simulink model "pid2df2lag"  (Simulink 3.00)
settings: Solver=ode45  SolverMode=SingleTasking  StartTime=0.0  StopTime=10.0  MaxStep=st_size  RelTol=1e-5  AbsTol=1e-6
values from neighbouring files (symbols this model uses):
  d_through_p = get(MAIN_MENU(19),'Value')    [cback.m]    (also in imcmenu.m = 0)
  Disturb = Setpoint    [mimo_MSF1DF_sim.m]    (also in mimo_MSF2DF_sim.m)
  Satlb = temp1    [cback.m]    (also in imcmenu.m = str2num(satlbs))
  Satub = temp1    [cback.m]    (also in imcmenu.m = str2num(satubs))
  Setpoint = zeros(1,n)    [mimo_MSF1DF_sim.m]    (also in mimo_MSF2DF_sim.m)
undefined symbols (not defined in the file or in its folder): a1, a2, b1, b2, denPd, denPs, keps, numPd, numPs, Pre_fil_den, Pre_fil_num
libraries: MIMO_lib x1

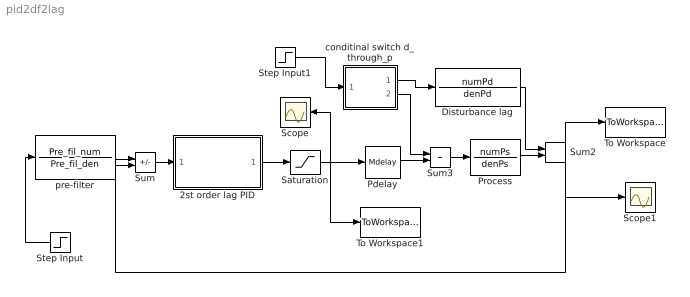
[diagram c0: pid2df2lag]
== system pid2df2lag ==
  2st order lag PID : Subsystem
  Disturbance lag : TransferFcn  Numerator=numPd  Denominator=denPd
  Pdelay : MIMO_lib/Mdelay  Mdelay=Pdelay
  Process : TransferFcn  Numerator=numPs  Denominator=denPs
  Saturation : Saturate  UpperLimit=Satub  LowerLimit=Satlb
  Scope : Scope
  Scope1 : Scope
  Step Input : Step  Orientation=left  Time=0  Before=0  After=Setpoint  SampleTime=0
  Step Input1 : Step  Time=0  Before=0  After=Disturb  SampleTime=0
  Sum : Sum  Inputs=+-  SaturateOnIntegerOverflow=on
  Sum2 : Sum  Inputs=++  SaturateOnIntegerOverflow=on
  Sum3 : Sum  Inputs=++  SaturateOnIntegerOverflow=on
  To Workspace : ToWorkspace  VariableName=simout  SampleTime=-1  SaveFormat=Matrix
  To Workspace1 : ToWorkspace  VariableName=effort  SampleTime=-1  SaveFormat=Matrix
  conditinal switch d_through_p : Subsystem  Description=pass input signal through out1 if condition is true.
  pre-filter : TransferFcn  Numerator=Pre_fil_num  Denominator=Pre_fil_den
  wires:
  Disturbance lag/1 -> Sum2/1
  Sum/1 -> 2st order lag PID/1(In1)
  pre-filter/1 -> Sum/1
  Step Input/1 -> pre-filter/1
  2st order lag PID/1(Out1) -> Saturation/1
  Step Input1/1 -> conditinal switch d_through_p/1(In)
  conditinal switch d_through_p/1(Out2) -> Disturbance lag/1
  conditinal switch d_through_p/2(Out1) -> Sum3/1
  Pdelay/1 -> Sum3/2
  Sum3/1 -> Process/1
  Process/1 -> Sum2/2
  Sum2/1 -> Sum/2, To Workspace/1, Scope1/1
  Saturation/1 -> Pdelay/1, Scope/1, To Workspace1/1

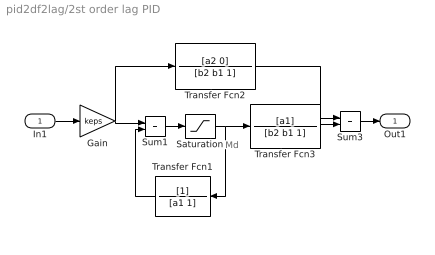
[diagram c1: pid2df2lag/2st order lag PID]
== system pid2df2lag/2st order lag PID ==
  note: Md
  In1 : Inport  Port=1  PortWidth=-1  SampleTime=-1  DataType=auto
  Gain : Gain  Gain=keps  SaturateOnIntegerOverflow=on
  Saturation : Saturate  UpperLimit=Satub  LowerLimit=Satlb
  Sum1 : Sum  Inputs=++  SaturateOnIntegerOverflow=on
  Sum3 : Sum  Inputs=++  SaturateOnIntegerOverflow=on
  Transfer Fcn1 : TransferFcn  Orientation=left  Numerator=[1]  Denominator=[a1 1]
  Transfer Fcn2 : TransferFcn  Numerator=[a2 0]  Denominator=[b2 b1 1]
  Transfer Fcn3 : TransferFcn  Numerator=[a1]  Denominator=[b2 b1 1]
  Out1 : Outport  Port=1  InitialOutput=0
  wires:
  Gain/1 -> Transfer Fcn2/1, Sum1/1
  Transfer Fcn1/1 -> Sum1/2
  Saturation/1 -> Transfer Fcn1/1, Transfer Fcn3/1
  Sum1/1 -> Saturation/1
  Transfer Fcn3/1 -> Sum3/2
  In1/1 -> Gain/1
  Sum3/1 -> Out1/1
  Transfer Fcn2/1 -> Sum3/1

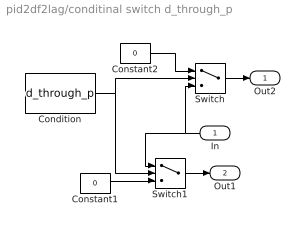
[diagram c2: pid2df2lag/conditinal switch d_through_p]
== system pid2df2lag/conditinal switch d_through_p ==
  In : Inport  Orientation=left  Port=1  PortWidth=-1  SampleTime=-1  DataType=auto
  Condition : Constant  Value=d_through_p
  Constant1 : Constant  Value=0
  Constant2 : Constant  Value=0
  Switch : Switch  Threshold=1
  Switch1 : Switch  Threshold=1
  Out2 : Outport  Port=1  InitialOutput=0
  Out1 : Outport  Port=2  InitialOutput=0
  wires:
  In/1 -> Switch/3, Switch1/1
  Condition/1 -> Switch1/2, Switch/2
  Constant1/1 -> Switch1/3
  Constant2/1 -> Switch/1
  Switch/1 -> Out2/1
  Switch1/1 -> Out1/1
